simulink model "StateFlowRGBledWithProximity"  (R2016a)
settings: Solver=FixedStepAuto  StartTime=0.0  StopTime=inf  RelTol=1e-3
libraries: miniQ x2

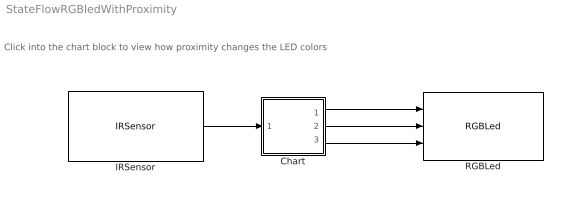
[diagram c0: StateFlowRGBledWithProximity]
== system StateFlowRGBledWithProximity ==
  note: Click into the chart block to view how proximity changes the LED colors
  Chart : Stateflow chart  TreatAsAtomicUnit=on
  IRSensor : miniQ/IRSensor  sampleTime_dd=0.01  debug_dd=off
  RGBLed : miniQ/RGBLed
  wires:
  IRSensor/1 -> Chart/1(prox)
  Chart/1(r) -> RGBLed/1
  Chart/2(g) -> RGBLed/2
  Chart/3(b) -> RGBLed/3

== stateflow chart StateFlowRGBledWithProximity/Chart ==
  state Green
    entry: r=0;
    g=255;
    b=0;
  state No object = green light [group]
  state Red
    entry: r = 255;
    g=0;
    b=0;
  state Object detected = red light [group]
  (default) -> Green
  Green -> Red : [prox>10]
  Red -> Green : [prox<10]
  data: prox input; r output; g output; b output
